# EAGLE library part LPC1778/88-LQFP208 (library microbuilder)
LPC1778/88 - ARM Cortex M3 - 120MHz, 512KB Flash, 96KB SRAM, 4KB EEPROM External Memory Controller LCD Controller 10/100 Ethernet USB 2.0 Host/Device/OTG 2 CAN 12-bit ADC 10-bit DAC SD/MMC I2S
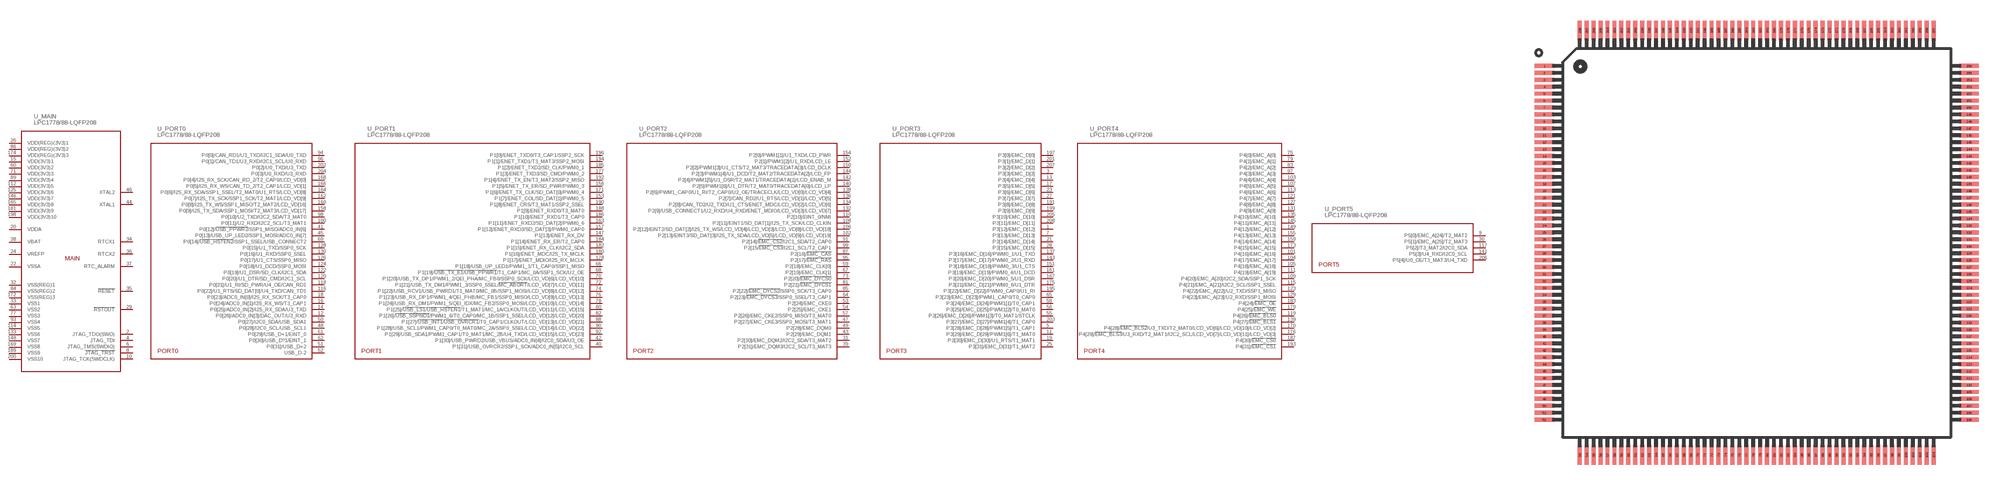
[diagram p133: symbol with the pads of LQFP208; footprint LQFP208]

Designator prefix U; gates _MAIN=LPC1788_PWR-208 _PORT0=LPC1788_PORT0-208 _PORT1=LPC1788_PORT1-208 _PORT2=LPC1788_PORT2-208 _PORT3=LPC1788_PORT3-208 _PORT4=LPC1788_PORT4-208 _PORT5=LPC1788_PORT5-208

## LPC1778/88-LQFP208  [LQFP208]
1  _PORT3:P3[12]/EMC_D[12]
2  _MAIN:JTAG_TDO(SWO)
3  _PORT3:P3[3]/EMC_D[3]
4  _MAIN:JTAG_TDI
5  _PORT3:P3[28]/EMC_D[28]/PWM1[5]/T1_CAP1
6  _MAIN:JTAG_TMS(SWDIO)
7  _PORT3:P3[13]/EMC_D[13]
8  _MAIN:!JTAG_TRST!
9  _PORT5:P5[0]/EMC_A[24]/T2_MAT2
10  _MAIN:JTAG_TCK(SWDCLK)
11  _PORT3:P3[29]/EMC_D[29]/PWM1[6]/T1_MAT0
12  _PORT0:P0[26]/ADC0_IN[3]/DAC_OUT/U3_RXD
13  _PORT3:P3[4]/EMC_D[4]
14  _PORT0:P0[25]/ADC0_IN[2]/I2S_RX_SDA/U3_TXD
15  _MAIN:VDD(3V3)1
16  _PORT0:P0[24]/ADC0_IN[1]/I2S_RX_WS/T3_CAP1
17  _PORT3:P3[5]/EMC_D[5]
18  _PORT0:P0[23]/ADC0_IN[0]/I2S_RX_SCK/T3_CAP0
19  _PORT3:P3[30]/EMC_D[30]/U1_RTS/T1_MAT1
20  _MAIN:VDDA
21  _PORT3:P3[14]/EMC_D[14]
22  _MAIN:VSSA
23  _PORT3:P3[6]/EMC_D[6]
24  _MAIN:VREFP
25  _PORT3:P3[31]/EMC_D[31]/T1_MAT2
26  _MAIN:VDD(REG)(3V3)1
27  _PORT3:P3[7]/EMC_D[7]
28  _PORT3:P3[15]/EMC_D[15]
29  _MAIN:!RSTOUT!
30  _PORT5:P5[1]/EMC_A[25]/T2_MAT3
31  _PORT2:P2[30]/EMC_DQM2/I2C2_SDA/T3_MAT2
32  _MAIN:VSS(REG)1
33  _MAIN:VSS1
34  _MAIN:RTCX1
35  _MAIN:!RESET!
36  _MAIN:RTCX2
37  _MAIN:RTC_ALARM
38  _MAIN:VBAT
39  _PORT2:P2[31]/EMC_DQM3/I2C2_SCL/T3_MAT3
40  _PORT1:P1[31]/USB_OVRCR2/SSP1_SCK/ADC0_IN[5]/I2C0_SCL
41  _PORT0:P0[12]/!USB_PPWR2!/SSP1_MISO/ADC0_IN[6]
42  _PORT1:P1[30]/USB_PWRD2/USB_VBUS/ADC0_IN[4]/I2C0_SDA/U3_OE
43  _PORT2:P2[29]/EMC_DQM1
44  _MAIN:XTAL1
45  _PORT0:P0[13]/USB_UP_LED2/SSP1_MOSI/ADC0_IN[7]
46  _MAIN:XTAL2
47  _PORT2:P2[27]/EMC_CKE3/SSP0_MOSI/T3_MAT1
48  _PORT0:P0[28]/I2C0_SCL/USB_SCL1
49  _PORT2:P2[28]/EMC_DQM0
50  _PORT0:P0[27]/I2C0_SDA/USB_SDA1
51  _PORT0:P0[31]/USB_D+2
52  _PORT0:USB_D-2
53  _PORT2:P2[24]/EMC_CKE0
54  _PORT2:P2[25]/EMC_CKE1
55  _PORT3:P3[26]/EMC_D[26]/PWM1[3]/T0_MAT1/STCLK
56  _PORT3:P3[25]/EMC_D[25]/PWM1[2]/T0_MAT0
57  _PORT2:P2[26]/EMC_CKE2/SSP0_MISO/T3_MAT0
58  _PORT3:P3[24]/EMC_D[24]/PWM1[1]/T0_CAP1
59  _PORT2:P2[18]/EMC_CLK[0]
60  _MAIN:VDD(3V3)2
61  _PORT0:P0[29]/USB_D+1/EINT_0
62  _PORT0:P0[30]/USB_D?1/EINT_1
63  _MAIN:VSS2
64  _PORT2:P2[23]/!EMC_DYCS3!/SSP0_SSEL/T3_CAP1
65  _PORT3:P3[23]/EMC_D[23]/PWM1_CAP0/T0_CAP0
66  _PORT1:P1[18]/USB_UP_LED1/PWM1_1/T1_CAP0/SSP1_MISO
67  _PORT2:P2[19]/EMC_CLK[1]
68  _PORT1:P1[19]/!USB_TX_E1!/!USB_PPWR1!/T1_CAP1/MC_0A/SSP1_SCK/U2_OE
69  _PORT0:P0[14]/!USB_HSTEN2!/SSP1_SSEL/USB_CONNECT2
70  _PORT1:P1[20]/USB_TX_DP1/PWM1_2/QEI_PHA/MC_FB0/SSP0_SCK/LCD_VD[6]/LCD_VD[10]
71  _MAIN:VDD(3V3)3
72  _PORT1:P1[21]/USB_TX_DM1/PWM1_3/SSP0_SSEL/!MC_ABORT!/LCD_VD[7]/LCD_VD[11]
73  _PORT2:P2[20]/!EMC_DYCS0!
74  _PORT1:P1[22]/USB_RCV1/USB_PWRD1/T1_MAT0/MC_0B/SSP1_MOSI/LCD_VD[8]/LCD_VD[12]
75  _PORT4:P4[0]/EMC_A[0]
76  _PORT1:P1[23]/USB_RX_DP1/PWM1_4/QEI_PHB/MC_FB1/SSP0_MISO/LCD_VD[9]/LCD_VD[13]
77  _MAIN:VSS3
78  _PORT1:P1[24]/USB_RX_DM1/PWM1_5/QEI_IDX/MC_FB2/SSP0_MOSI/LCD_VD[10]/LCD_VD[14]
79  _PORT4:P4[1]/EMC_A[1]
80  _PORT1:P1[25]/!USB_LS1!/!USB_HSTEN1!/T1_MAT1/MC_1A/CLKOUT/LCD_VD[11]/LCD_VD[15]
81  _PORT2:P2[21]/!EMC_DYCS1!
82  _PORT1:P1[26]/!USB_SSPND1!/PWM1_6/T0_CAP0/MC_1B/SSP1_SSEL/LCD_VD[12]/LCD_VD[20]
83  _PORT4:P4[2]/EMC_A[2]
84  _MAIN:VSS(REG)2
85  _PORT2:P2[22]/!EMC_DYCS2!/SSP0_SCK/T3_CAP0
86  _MAIN:VDD(REG)(3V3)2
87  _PORT2:P2[16]/!EMC_CAS!
88  _PORT1:P1[27]/!USB_INT1!/!USB_OVRCR1!/T0_CAP1/CLKOUT/LCD_VD[13]/LCD_VD[21]
89  _MAIN:VDD(3V3)4
90  _PORT1:P1[28]/USB_SCL1/PWM1_CAP0/T0_MAT0/MC_2A/SSP0_SSEL/LCD_VD[14]/LCD_VD[22]
91  _PORT2:P2[14]/!EMC_CS2!/I2C1_SDA/T2_CAP0
92  _PORT1:P1[29]/USB_SDA1/PWM1_CAP1/T0_MAT1/MC_2B/U4_TXD/LCD_VD[15]/LCD_VD[23]
93  _MAIN:VSS4
94  _PORT0:P0[0]/CAN_RD1/U3_TXD/I2C1_SDA/U0_TXD
95  _PORT2:P2[17]/!EMC_RAS!
96  _PORT0:P0[1]/CAN_TD1/U3_RXD/I2C1_SCL/U0_RXD
97  _PORT4:P4[3]/EMC_A[3]
98  _PORT0:P0[10]/U2_TXD/I2C2_SDA/T3_MAT0
99  _PORT2:P2[15/!EMC_CS3!/I2C1_SCL/T2_CAP1
100  _PORT0:P0[11]/U2_RXD/I2C2_SCL/T3_MAT1
101  _PORT4:P4[16]/EMC_A[16]
102  _PORT2:P2[13]/EINT3/SD_DAT[3]/I2S_TX_SDA/LCD_VD[5]/LCD_VD[9]/LCD_VD[19]
103  _PORT4:P4[4]/EMC_A[4]
104  _PORT4:P4[17]/EMC_A[17]
105  _PORT4:P4[18]/EMC_A[18]
106  _PORT2:P2[12]/EINT2/SD_DAT[2]/I2S_TX_WS/LCD_VD[4]/LCD_VD[3]/LCD_VD[8]/LCD_VD[18]
107  _PORT4:P4[5]/EMC_A[5]
108  _PORT2:P2[11]/EINT1/SD_DAT[1]/I2S_TX_SCK/LCD_CLKIN
109  _PORT4:P4[20]/EMC_A[20]/I2C2_SDA/SSP1_SCK
110  _PORT2:P2[10]/EINT_0/NMI
111  _PORT4:P4[19]/EMC_A[19]
112  _MAIN:VDD(3V3)5
113  _PORT4:P4[6]/EMC_A[6]
114  _MAIN:VSS5
115  _PORT4:P4[21]/EMC_A[21]/I2C2_SCL/SSP1_SSEL
116  _PORT0:P0[22]/U1_RTS/SD_DAT[0]/U4_TXD/CAN_TD1
117  _PORT5:P5[2]/T3_MAT2/I2C0_SDA
118  _PORT0:P0[21]/U1_RI/SD_PWR/U4_OE/CAN_RD1
119  _PORT4:P4[26]/!EMC_BLS0!
120  _PORT0:P0[20]/U1_DTR/SD_CMD/I2C1_SCL
121  _PORT4:P4[7]/EMC_A[7]
122  _PORT0:P0[19]/U1_DSR/SD_CLK/I2C1_SDA
123  _PORT4:P4[22]/EMC_A[22]/U2_TXD/SSP1_MISO
124  _PORT0:P0[18]/U1_DCD/SSP0_MOSI
125  _MAIN:VDD(3V3)6
126  _PORT0:P0[17]/U1_CTS/SSP0_MISO
127  _PORT4:P4[8]/EMC_A[8]
128  _PORT0:P0[15]/U1_TXD/SSP0_SCK
129  _PORT4:P4[23]/EMC_A[23]/U2_RXD/SSP1_MOSI
130  _PORT0:P0[16]/U1_RXD/SSP0_SSEL
131  _PORT4:P4[9]/EMC_A[9]
132  _PORT2:P2[9]/USB_CONNECT1/U2_RXD/U4_RXD/ENET_MDIO/LCD_VD[3]/LCD_VD[7]
133  _MAIN:VSS6
134  _PORT2:P2[8]/CAN_TD2/U2_TXD/U1_CTS/ENET_MDC/LCD_VD[2]/LCD_VD[6]
135  _PORT4:P4[10]/EMC_A[10]
136  _PORT2:P2[7]/CAN_RD2/U1_RTS/LCD_VD[1]/LCD_VD[5]
137  _PORT3:P3[16]/EMC_D[16]/PWM0_1/U1_TXD
138  _PORT2:P2[6]/PWM1_CAP0/U1_RI/T2_CAP0/U2_OE/TRACECLK/LCD_VD[0]/LCD_VD[4]
139  _PORT4:P4[27]/!EMC_BLS1!
140  _PORT2:P2[5]/PWM1[6]/U1_DTR/T2_MAT0/TRACEDATA[0]/LCD_LP
141  _PORT5:P5[3]/U4_RXD/I2C0_SCL
142  _PORT2:P2[4]/PWM1[5]/U1_DSR/T2_MAT1/TRACEDATA[1]/LCD_ENAB_M
143  _PORT3:P3[17]/EMC_D[17]/PWM0_2/U1_RXD
144  _PORT2:P2[3]/PWM1[4]/U1_DCD/T2_MAT2/TRACEDATA[2]/LCD_FP
145  _PORT4:P4[11]/EMC_A[11]
146  _MAIN:VDD(3V3)7
147  _PORT1:P1[13]/ENET_RX_DV
148  _MAIN:VSS7
149  _PORT4:P4[12]/EMC_A[12]
150  _PORT2:P2[2]/PWM1[3]/U1_CTS/T2_MAT3/TRACEDATA[3]/LCD_DCLK
151  _PORT3:P3[18]/EMC_D[18]/PWM0_3/U1_CTS
152  _PORT2:P2[1]/PWM1[2]/U1_RXD/LCD_LE
153  _PORT1:P1[7]/ENET_COL/SD_DAT[1]/PWM0_5
154  _PORT2:P2[0]/PWM1[1]/U1_TXD/LCD_PWR
155  _PORT4:P4[13]/EMC_A[13]
156  _PORT1:P1[5]/ENET_TX_ER/SD_PWR/PWM0_3
157  _PORT1:P1[12]/ENET_RXD3/SD_DAT[3]/PWM0_CAP0
158  _PORT0:P0[9]/I2S_TX_SDA/SSP1_MOSI/T2_MAT3/LCD_VD[17]
159  _PORT4:P4[14]/EMC_A[14]
160  _PORT0:P0[8]/I2S_TX_WS/SSP1_MISO/T2_MAT2/LCD_VD[16]
161  _PORT3:P3[19]/EMC_D[19]/PWM0_4/U1_DCD
162  _PORT0:P0[7]/I2S_TX_SCK/SSP1_SCK/T2_MAT1/LCD_VD[9]
163  _PORT1:P1[11]/ENET_RXD2/SD_DAT[2]/PWM0_6
164  _PORT0:P0[6]/I2S_RX_SDA/SSP1_SSEL/T2_MAT0/U1_RTS/LCD_VD[8]
165  _MAIN:VDD(3V3)8
166  _PORT0:P0[5]/I2S_RX_WS/CAN_TD_2/T2_CAP1/LCD_VD[1]
167  _PORT3:P3[20]/EMC_D[20]/PWM0_5/U1_DSR
168  _PORT0:P0[4]/I2S_RX_SCK/CAN_RD_2/T2_CAP0/LCD_VD[0]
169  _MAIN:VSS8
170  _PORT4:P4[28]/!EMC_BLS2!/U3_TXD/T2_MAT0/LCD_VD[6]/LCD_VD[10]/LCD_VD[2]
171  _PORT1:P1[6]/ENET_TX_CLK/SD_DAT[0]/PWM0_4
172  _MAIN:VSS(REG)3
173  _PORT4:P4[15]/EMC_A[15]
174  _MAIN:VDD(REG)(3V3)3
175  _PORT3:P3[21]/EMC_D[21]/PWM0_6/U1_DTR
176  _PORT4:P4[29]/!EMC_BLS3!/U3_RXD/T2_MAT1/I2C2_SCL/LCD_VD[7]/LCD_VD[11]/LCD_VD[3]
177  _PORT1:P1[3]/ENET_TXD3/SD_CMD/PWM0_2
178  _PORT1:P1[17]/ENET_MDIO/I2S_RX_MCLK
179  _PORT4:P4[25]/!EMC_WE!
180  _PORT1:P1[16]/ENET_MDC/I2S_TX_MCLK
181  _MAIN:VDD(3V3)9
182  _PORT1:P1[15]/ENET_RX_CLK/I2C2_SDA
183  _PORT4:P4[24]/!EMC_OE!
184  _PORT1:P1[14]/ENET_RX_ER/T2_CAP0
185  _PORT1:P1[2]/ENET_TXD2/SD_CLK/PWM0_1
186  _PORT1:P1[10]/ENET_RXD1/T3_CAP0
187  _PORT4:P4[30]/!EMC_CS0!
188  _PORT1:P1[9]/ENET_RXD0/T3_MAT0
189  _MAIN:VSS9
190  _PORT1:P1[8]/ENET_CRS/T3_MAT1/SSP2_SSEL
191  _PORT3:P3[8]/EMC_D[8]
192  _PORT1:P1[4]/ENET_TX_EN/T3_MAT2/SSP2_MISO
193  _PORT4:P4[31]/!EMC_CS1!
194  _PORT1:P1[1]/ENET_TXD1/T3_MAT3/SSP2_MOSI
195  _PORT3:P3[22]/EMC_D[22]/PWM0_CAP0/U1_RI
196  _PORT1:P1[0]/ENET_TXD0/T3_CAP1/SSP2_SCK
197  _PORT3:P3[0]/EMC_D[0]
198  _MAIN:VDD(3V3)10
199  _PORT3:P3[9]/EMC_D[9]
200  _MAIN:VSS10
201  _PORT3:P3[1]/EMC_D[1]
202  _PORT0:P0[2]/U0_TXD/U3_TXD
203  _PORT3:P3[27]/EMC_D[27]/PWM1[4]/T1_CAP0
204  _PORT0:P0[3]/U0_RXD/U3_RXD
205  _PORT3:P3[10]/EMC_D[10]
206  _PORT5:P5[4]/U0_OE/T3_MAT3/U4_TXD
207  _PORT3:P3[2]/EMC_D[2]
208  _PORT3:P3[11]/EMC_D[11]

## Footprint LQFP208 (pad centres in mm)
smd 1.4 x 0.29: 1 -15.3,12.75; 2 -15.3,12.25; 3 -15.3,11.75; 4 -15.3,11.25; 5 -15.3,10.75; 6 -15.3,10.25; 7 -15.3,9.75; 8 -15.3,9.25; 9 -15.3,8.75; 10 -15.3,8.25; 11 -15.3,7.75; 12 -15.3,7.25; 13 -15.3,6.75; 14 -15.3,6.25; 15 -15.3,5.75; 16 -15.3,5.25; 17 -15.3,4.75; 18 -15.3,4.25; 19 -15.3,3.75; 20 -15.3,3.25; 21 -15.3,2.75; 22 -15.3,2.25; 23 -15.3,1.75; 24 -15.3,1.25; 25 -15.3,0.75; 26 -15.3,0.25; 27 -15.3,-0.25; 28 -15.3,-0.75; 29 -15.3,-1.25; 30 -15.3,-1.75; 31 -15.3,-2.25; 32 -15.3,-2.75; 33 -15.3,-3.25; 34 -15.3,-3.75; 35 -15.3,-4.25; 36 -15.3,-4.75; 37 -15.3,-5.25; 38 -15.3,-5.75; 39 -15.3,-6.25; 40 -15.3,-6.75; 41 -15.3,-7.25; 42 -15.3,-7.75; 43 -15.3,-8.25; 44 -15.3,-8.75; 45 -15.3,-9.25; 46 -15.3,-9.75; 47 -15.3,-10.25; 48 -15.3,-10.75; 49 -15.3,-11.25; 50 -15.3,-11.75; 51 -15.3,-12.25; 52 -15.3,-12.75; 105 15.3,-12.75; 106 15.3,-12.25; 107 15.3,-11.75; 108 15.3,-11.25; 109 15.3,-10.75; 110 15.3,-10.25; 111 15.3,-9.75; 112 15.3,-9.25; 113 15.3,-8.75; 114 15.3,-8.25; 115 15.3,-7.75; 116 15.3,-7.25; 117 15.3,-6.75; 118 15.3,-6.25; 119 15.3,-5.75; 120 15.3,-5.25; 121 15.3,-4.75; 122 15.3,-4.25; 123 15.3,-3.75; 124 15.3,-3.25; 125 15.3,-2.75; 126 15.3,-2.25; 127 15.3,-1.75; 128 15.3,-1.25; 129 15.3,-0.75; 130 15.3,-0.25; 131 15.3,0.25; 132 15.3,0.75; 133 15.3,1.25; 134 15.3,1.75; 135 15.3,2.25; 136 15.3,2.75; 137 15.3,3.25; 138 15.3,3.75; 139 15.3,4.25; 140 15.3,4.75; 141 15.3,5.25; 142 15.3,5.75; 143 15.3,6.25; 144 15.3,6.75; 145 15.3,7.25; 146 15.3,7.75; 147 15.3,8.25; 148 15.3,8.75; 149 15.3,9.25; 150 15.3,9.75; 151 15.3,10.25; 152 15.3,10.75; 153 15.3,11.25; 154 15.3,11.75; 155 15.3,12.25; 156 15.3,12.75
smd 0.29 x 1.4: 53 -12.75,-15.3; 54 -12.25,-15.3; 55 -11.75,-15.3; 56 -11.25,-15.3; 57 -10.75,-15.3; 58 -10.25,-15.3; 59 -9.75,-15.3; 60 -9.25,-15.3; 61 -8.75,-15.3; 62 -8.25,-15.3; 63 -7.75,-15.3; 64 -7.25,-15.3; 65 -6.75,-15.3; 66 -6.25,-15.3; 67 -5.75,-15.3; 68 -5.25,-15.3; 69 -4.75,-15.3; 70 -4.25,-15.3; 71 -3.75,-15.3; 72 -3.25,-15.3; 73 -2.75,-15.3; 74 -2.25,-15.3; 75 -1.75,-15.3; 76 -1.25,-15.3; 77 -0.75,-15.3; 78 -0.25,-15.3; 79 0.25,-15.3; 80 0.75,-15.3; 81 1.25,-15.3; 82 1.75,-15.3; 83 2.25,-15.3; 84 2.75,-15.3; 85 3.25,-15.3; 86 3.75,-15.3; 87 4.25,-15.3; 88 4.75,-15.3; 89 5.25,-15.3; 90 5.75,-15.3; 91 6.25,-15.3; 92 6.75,-15.3; 93 7.25,-15.3; 94 7.75,-15.3; 95 8.25,-15.3; 96 8.75,-15.3; 97 9.25,-15.3; 98 9.75,-15.3; 99 10.25,-15.3; 100 10.75,-15.3; 101 11.25,-15.3; 102 11.75,-15.3; 103 12.25,-15.3; 104 12.75,-15.3; 157 12.75,15.3; 158 12.25,15.3; 159 11.75,15.3; 160 11.25,15.3; 161 10.75,15.3; 162 10.25,15.3; 163 9.75,15.3; 164 9.25,15.3; 165 8.75,15.3; 166 8.25,15.3; 167 7.75,15.3; 168 7.25,15.3; 169 6.75,15.3; 170 6.25,15.3; 171 5.75,15.3; 172 5.25,15.3; 173 4.75,15.3; 174 4.25,15.3; 175 3.75,15.3; 176 3.25,15.3; 177 2.75,15.3; 178 2.25,15.3; 179 1.75,15.3; 180 1.25,15.3; 181 0.75,15.3; 182 0.25,15.3; 183 -0.25,15.3; 184 -0.75,15.3; 185 -1.25,15.3; 186 -1.75,15.3; 187 -2.25,15.3; 188 -2.75,15.3; 189 -3.25,15.3; 190 -3.75,15.3; 191 -4.25,15.3; 192 -4.75,15.3; 193 -5.25,15.3; 194 -5.75,15.3; 195 -6.25,15.3; 196 -6.75,15.3; 197 -7.25,15.3; 198 -7.75,15.3; 199 -8.25,15.3; 200 -8.75,15.3; 201 -9.25,15.3; 202 -9.75,15.3; 203 -10.25,15.3; 204 -10.75,15.3; 205 -11.25,15.3; 206 -11.75,15.3; 207 -12.25,15.3; 208 -12.75,15.3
